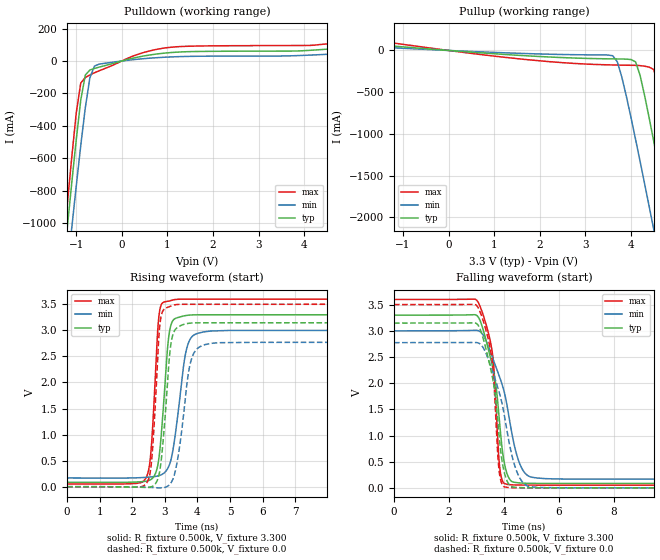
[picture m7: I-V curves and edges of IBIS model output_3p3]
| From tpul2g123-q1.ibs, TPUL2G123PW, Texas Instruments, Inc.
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|   Model output_3p3
[Model] output_3p3
Model_type Output
Polarity   Non-Inverting
Enable   Active-High
Vmeas = 3.3v
Cref = 15pf
C_comp   2.098pF   1.863pF   2.341pF
[Temperature Range]   27.000   0.125k   -40.000
[Voltage Range]   3.300V   3.000V   3.600V
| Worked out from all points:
|   slope of the pulldown table from 0 to 0.495 V, typ, clamps not added: 15.7 ohm
|   slope of the pullup table from 0 to 0.495 V, typ, clamps not added: 24.5 ohm
|   rising waveform, R_fixture 0.500k, V_fixture 3.300: 20-80 % time 233ps typ, 345ps min, 187ps max; typ from 0.084 V to 3.3 V
|   rising waveform, R_fixture 0.500k, V_fixture 0.0: 20-80 % time 236ps typ, 334ps min, 189ps max; typ from 0 V to 3.15 V
|   falling waveform, R_fixture 0.500k, V_fixture 3.300: 20-80 % time 512ps typ, 791ps min, 326ps max; typ from 3.3 V to 0.084 V
|   falling waveform, R_fixture 0.500k, V_fixture 0.0: 20-80 % time 491ps typ, 734ps min, 320ps max; typ from 3.15 V to 0 V
[Pulldown]
|Voltage   I(typ)   I(min)   I(max)
-3.3V     -6.285A    -5.959A    -6.676A
-1.3V     -1.325A    -1.574A    -1.201A
-1.2V     -1.039A    -1.303A    -897.8mA
-1.1V     -758.3mA   -1.035A    -601.5mA
-1V       -487.8mA   -773.2mA   -322.7mA
-900mV    -241.1mA   -521mA     -135.5mA
-800mV    -86.65mA   -287.6mA   -101.5mA
-700mV    -55.58mA   -103.7mA   -86.11mA
-500mV    -37.94mA   -19.6mA    -60.66mA
1V        50.23mA    24.09mA    82.34mA
4.2V      67.13mA    37.23mA    97.17mA
6.6V      132.1mA    38.3mA     193.1mA
[Pullup]
|Voltage   I(typ)   I(min)   I(max)
-3.3V     144.9mA    87.19mA    244.7mA
3.6V      -101mA     -63.35mA   -173.8mA
3.7V      -101.7mA   -135.1mA   -174.9mA
4V        -108.6mA   -802.6mA   -177.7mA
4.1V      -136.4mA   -1.063A    -178.6mA
4.2V      -297.8mA   -1.329A    -181.7mA
4.5V      -1.089A    -2.147A    -229.5mA
4.8V      -1.951A    -2.976A    -998.4mA
4.9V      -2.242A    -3.245A    -1.3A
5.1V      -2.829A    -3.705A    -1.913A
5.2V      -3.123A    -3.903A    -2.223A
6.6V      -6.322A    -6.531A    -6.117A
[Ramp]
| variable   typ   min   max
dV/dt_r   1.889/0.236n   1.665/0.334n   2.102/0.189n
dV/dt_f   1.930/0.513n   1.700/0.790n   2.129/0.326n
R_load = 0.500k
[Rising Waveform]
R_fixture= 0.500k
V_fixture= 3.300
V_fixture_min= 3.000
V_fixture_max= 3.600
|time   V(typ)   V(min)   V(max)
0s        83.91mV    167.2mV    52.25mV
2.42ns    105.1mV    179.5mV    167.1mV
2.577ns   139.9mV    187.7mV    706.1mV
2.779ns   400.4mV    205.7mV    2.983V
2.843ns   684.9mV    217mV      3.388V
3.116ns   2.864V     385.9mV    3.562V
3.332ns   3.233V     1.057V     3.594V
3.698ns   3.29V      2.715V     3.599V
4.398ns   3.3V       2.987V     3.6V
50ns      3.3V       3V         3.6V
[Rising Waveform]
R_fixture= 0.500k
V_fixture= 0.0
V_fixture_min= 0.0
V_fixture_max= 0.0
|time   V(typ)   V(min)   V(max)
0s        604.7nV    437.8nV    1.524uV
2.464ns   -12.76mV   -11.5mV    91.96mV
2.603ns   2.889mV    -15.19mV   566.6mV
2.865ns   393.4mV    -22.16mV   3.197V
3.162ns   2.623V     53.21mV    3.461V
3.34ns    3.031V     356.7mV    3.494V
3.705ns   3.134V     2.109V     3.5V
3.845ns   3.142V     2.502V     3.501V
4.645ns   3.146V     2.763V     3.501V
50ns      3.149V     2.775V     3.502V
[Falling Waveform]
R_fixture= 0.500k
V_fixture= 3.300
V_fixture_min= 3.000
V_fixture_max= 3.600
|time   V(typ)   V(min)   V(max)
0s        3.3V       3V         3.6V
3.036ns   3.284V     3.008V     3.568V
3.542ns   2.415V     2.552V     2.702V
3.647ns   2.16V      2.4V       2.205V
3.854ns   1.18V      2.101V     361.3mV
3.988ns   555.3mV    1.879V     93.82mV
4.158ns   211.9mV    1.439V     64.71mV
4.655ns   91.15mV    369.1mV    53.39mV
5.501ns   84.37mV    176.1mV    52.36mV
50ns      83.91mV    167.2mV    52.25mV
[Falling Waveform]
R_fixture= 0.500k
V_fixture= 0.0
V_fixture_min= 0.0
V_fixture_max= 0.0
|time   V(typ)   V(min)   V(max)
0s        3.149V     2.775V     3.502V
3.059ns   3.111V     2.77V      3.447V
3.549ns   2.198V     2.282V     2.521V
3.626ns   1.985V     2.162V     2.108V
3.827ns   983.3mV    1.828V     320.8mV
3.946ns   469.3mV    1.577V     55.2mV
4.109ns   139.3mV    1.101V     10.4mV
4.629ns   4.056mV    142.8mV    547.7uV
5.381ns   304.2uV    5.876mV    97.39uV
50ns      642.9nV    3.008uV    123.7nV
